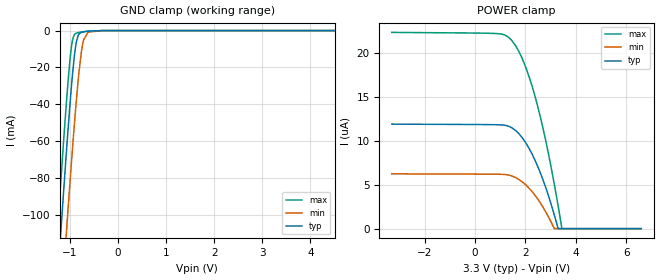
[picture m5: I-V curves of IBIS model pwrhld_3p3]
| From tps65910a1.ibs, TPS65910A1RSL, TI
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|   pwrhld_3p3 Model
[Model]   pwrhld_3p3
Model_type   Input
Vinl = 0.45
Vinh = 1.3
|   typ   min   max
|   (nom PVT)   (fast PVT)   (slow PVT)
C_comp   1.631e-13   1.628e-13   1.641e-13
| Where nom  PVT is Nominal Process, 3.3V, 27C
|   Fast PVT is Strong Process,  3.45V, -40C
|   Slow PVT is Weak Process,   3.15V, 125C
[Voltage Range]   3.3   3.15   3.45
|Junction Temperature
[Temperature Range]   27   125   -40
[Power Clamp Reference]   3.3   3.15   3.45
[GND Clamp Reference]   0   0   0
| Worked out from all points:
|   GND clamp passes 1 mA (typ) near -0.76 V on its own axis
[GND Clamp]
|   Voltage   I(typ)   I(min)   I(max)
-3.3V     -980.1mA   -1.019A    -957.7mA
-1.254V   -135.5mA   -179.7mA   -108mA
-1.223V   -123.4mA   -167.7mA   -95.9mA
-1.13V    -87.83mA   -131.9mA   -60.48mA
-1.067V   -64.51mA   -108.1mA   -37.83mA
-966.9mV  -30.7mA    -71.98mA   -9.039mA
-936.7mV  -21.85mA   -61.56mA   -4.402mA
-868.2mV  -6.838mA   -39.27mA   -1.428mA
-809.1mV  -1.861mA   -22.57mA   -1.035mA
-735.9mV  -755.4uA   -7.83mA    -721.2uA
-619.3mV  -342.2uA   -826.2uA   -313uA
6.6V      0A         0A         0A
[POWER Clamp]
|   Voltage   I(typ)   I(min)   I(max)
-3.3V     11.91uA    6.246uA    22.36uA
808.9mV   11.84uA    6.203uA    22.24uA
1.309V    11.7uA     6.122uA    21.85uA
1.606V    11.2uA     5.829uA    20.87uA
1.841V    10.48uA    5.407uA    19.6uA
2.079V    9.485uA    4.811uA    17.89uA
2.379V    7.822uA    3.812uA    15.12uA
2.833V    4.47uA     1.784uA    9.685uA
3.148V    1.567uA    11.93nA    5.064uA
3.297V    35.17nA    0A         2.647uA
3.455V    0A         0A         0A
6.6V      0A         0A         0A
